FUNCTION_BLOCK FB_LN_IED_LD1_LLN0 EXTENDS FB_AcsiCommonLogicalNodeClass
VAR_INPUT
	NamPlt: FB_DO_IED_LD1_LLN0_NamPlt := (sClass:='LPL', bLinkResult:=THIS^.AddDataToContainer(ipData:=NamPlt));
	Beh: FB_DO_IED_LD1_LLN0_Beh := (sClass:='ENS', bLinkResult:=THIS^.AddDataToContainer(ipData:=Beh));
	Health: FB_DO_IED_LD1_LLN0_Health := (sClass:='ENS', bLinkResult:=THIS^.AddDataToContainer(ipData:=Health));
	Mod_: FB_DO_IED_LD1_LLN0_Mod := (sObjectName:='Mod', sClass:='ENC', bLinkResult:=THIS^.AddDataToContainer(ipData:=Mod_));
	
	DS1: FB_DS_IED_LD1_LLN0_DS1 := (bLinkResult:=THIS^.AddDataSetToContainer(ipDataSet:=DS1));
	DS2: FB_DS_IED_LD1_LLN0_DS2 := (bLinkResult:=THIS^.AddDataSetToContainer(ipDataSet:=DS2));
	DS3: FB_DS_IED_LD1_LLN0_DS3 := (bLinkResult:=THIS^.AddDataSetToContainer(ipDataSet:=DS3));
	
	urcb101: FB_ScsmUrCBImplClass := (RptID:=(sValue:='IEDLD1/LLN0.urcb101'), DatSet:=(sValue:='IEDLD1/LLN0.DS1'), ConfRev:=(nValue:=1), OptFlds:=(SequenceNumber:=TRUE, ReportTimeStamp:=TRUE, ReasonForInclusion:=TRUE, DataSetName:=TRUE, DataReference:=TRUE, BufferOverflow:=FALSE, EntryID:=FALSE, ConfRevision:=TRUE), TrgOps:=(DataChange:=TRUE, QualityChange:=TRUE, DataUpdate:=FALSE, Integrity:=TRUE, GeneralInterrogation:=TRUE), IntgPd:=(nValue:=2000), bLinkResult:=THIS^.AddUnbufferedReportControlBlockToContainer(ipUnbufferedReportControlBlock:=urcb101));
	urcb201: FB_ScsmUrCBImplClass := (RptID:=(sValue:='IEDLD1/LLN0.urcb201'), DatSet:=(sValue:='IEDLD1/LLN0.DS2'), ConfRev:=(nValue:=1), OptFlds:=(SequenceNumber:=TRUE, ReportTimeStamp:=TRUE, ReasonForInclusion:=TRUE, DataSetName:=TRUE, DataReference:=FALSE, BufferOverflow:=FALSE, EntryID:=FALSE, ConfRevision:=TRUE), TrgOps:=(DataChange:=TRUE, QualityChange:=TRUE, DataUpdate:=TRUE, Integrity:=TRUE, GeneralInterrogation:=TRUE), IntgPd:=(nValue:=5000), bLinkResult:=THIS^.AddUnbufferedReportControlBlockToContainer(ipUnbufferedReportControlBlock:=urcb201));
	urcb301: FB_ScsmUrCBImplClass := (RptID:=(sValue:='IEDLD1/LLN0.urcb301'), DatSet:=(sValue:='IEDLD1/LLN0.DS3'), ConfRev:=(nValue:=1), OptFlds:=(SequenceNumber:=TRUE, ReportTimeStamp:=TRUE, ReasonForInclusion:=TRUE, DataSetName:=TRUE, DataReference:=FALSE, BufferOverflow:=FALSE, EntryID:=FALSE, ConfRevision:=TRUE), TrgOps:=(DataChange:=TRUE, QualityChange:=TRUE, DataUpdate:=TRUE, Integrity:=TRUE, GeneralInterrogation:=TRUE), IntgPd:=(nValue:=5000), bLinkResult:=THIS^.AddUnbufferedReportControlBlockToContainer(ipUnbufferedReportControlBlock:=urcb301));
	brcb101: FB_ScsmBrCBImplClass := (RptID:=(sValue:='IEDLD1/LLN0.brcb101'), DatSet:=(sValue:='IEDLD1/LLN0.DS1'), ConfRev:=(nValue:=1), OptFlds:=(SequenceNumber:=TRUE, ReportTimeStamp:=TRUE, ReasonForInclusion:=TRUE, DataSetName:=TRUE, DataReference:=TRUE, BufferOverflow:=TRUE, EntryID:=TRUE, ConfRevision:=TRUE), TrgOps:=(DataChange:=TRUE, QualityChange:=TRUE, DataUpdate:=FALSE, Integrity:=TRUE, GeneralInterrogation:=TRUE), IntgPd:=(nValue:=2000), bLinkResult:=THIS^.AddBufferedReportControlBlockToContainer(ipBufferedReportControlBlock:=brcb101));
	brcb201: FB_ScsmBrCBImplClass := (RptID:=(sValue:='IEDLD1/LLN0.brcb201'), DatSet:=(sValue:='IEDLD1/LLN0.DS2'), ConfRev:=(nValue:=1), OptFlds:=(SequenceNumber:=TRUE, ReportTimeStamp:=TRUE, ReasonForInclusion:=TRUE, DataSetName:=TRUE, DataReference:=FALSE, BufferOverflow:=TRUE, EntryID:=TRUE, ConfRevision:=TRUE), TrgOps:=(DataChange:=TRUE, QualityChange:=TRUE, DataUpdate:=TRUE, Integrity:=TRUE, GeneralInterrogation:=TRUE), IntgPd:=(nValue:=5000), bLinkResult:=THIS^.AddBufferedReportControlBlockToContainer(ipBufferedReportControlBlock:=brcb201));
	brcb301: FB_ScsmBrCBImplClass := (RptID:=(sValue:='IEDLD1/LLN0.brcb301'), DatSet:=(sValue:='IEDLD1/LLN0.DS3'), ConfRev:=(nValue:=1), OptFlds:=(SequenceNumber:=TRUE, ReportTimeStamp:=TRUE, ReasonForInclusion:=TRUE, DataSetName:=TRUE, DataReference:=FALSE, BufferOverflow:=TRUE, EntryID:=TRUE, ConfRevision:=TRUE), TrgOps:=(DataChange:=TRUE, QualityChange:=TRUE, DataUpdate:=TRUE, Integrity:=TRUE, GeneralInterrogation:=TRUE), IntgPd:=(nValue:=5000), bLinkResult:=THIS^.AddBufferedReportControlBlockToContainer(ipBufferedReportControlBlock:=brcb301));
END_VAR
VAR
END_VAR

END_FUNCTION_BLOCK
